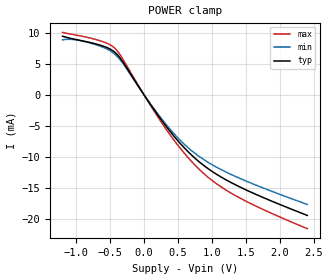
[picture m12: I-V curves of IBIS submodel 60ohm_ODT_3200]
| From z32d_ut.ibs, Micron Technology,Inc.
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| SUBMODEL 60ohm_ODT_3200
[Submodel]   60ohm_ODT_3200
Submodel_type  Dynamic_clamp
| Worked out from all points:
|   POWER clamp passes 1 mA (typ) near -0.06 V on its own axis
[POWER Clamp]
|   Voltage   I(typ)   I(min)   I(max)
-1.2V     9.457mA    8.874mA    10.08mA
-1.035V   9.006mA    8.917mA    9.714mA
-780mV    8.409mA    8.326mA    9.136mA
-540mV    7.603mA    7.368mA    8.296mA
-415mV    6.72mA     6.403mA    7.359mA
-315mV    5.383mA    5.135mA    5.811mA
110mV     -1.785mA   -1.69mA    -1.944mA
400mV     -6.107mA   -5.739mA   -6.686mA
695mV     -9.64mA    -8.936mA   -10.66mA
940mV     -11.85mA   -10.84mA   -13.24mA
1.455V    -15.06mA   -13.65mA   -16.86mA
2.4V      -19.39mA   -17.62mA   -21.52mA
